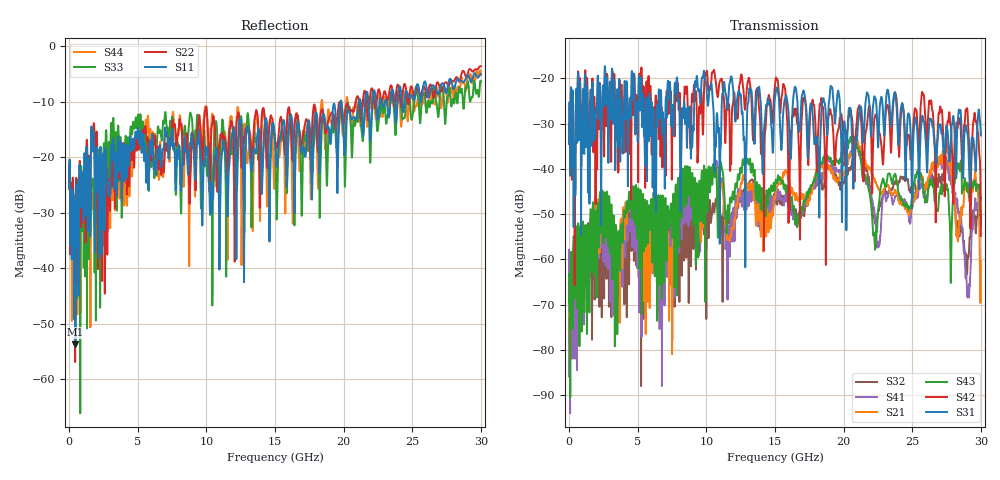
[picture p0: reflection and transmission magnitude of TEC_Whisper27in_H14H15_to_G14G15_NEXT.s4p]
! Tyco Electronics
! H14F15-H14G15_NEXT
!! PART DESCRIPTION: Whisper 27in Megtron 6 VLP-HVLP-VLP Channel Model, bulkhead 2.4mm test pts
!! MODEL DESCRIPTION: System 4-port S-parameter
!! MODEL STATUS: Measured
!! MODEL GEOMETRY: Channel Model
!! MODEL FREQUENCY RANGE: DC to 30.000 GHz in 10.000 MHz frequency steps
!! MODEL EDGE RATE LIMITATION: 12.500 ps (Using conservative 0.5/Fmax rule of thumb)
!! TIME-DOMAIN TRANSFORM CAUTIONS:
!! 1.) Do not simulate transient edge rates faster than the number listed above.  Edge rates faster than this number
!!  contain significant spectral content at frequencies above the model's highest frequency.
!! 2.) Even when simulating edge rates that are slower than the number listed above, be aware that the best time
!!  resolution possible with a direct iFFT is (1 / 2Fmax).  As a result, time resolution is typically not adequate
!!  for most time-domain simulations unless tricks such as windowing are used to minimize leakage and aliasing.
!! 3.) Because the model has a uniform frequency step, a direct iFFT will result in an impulse that that has a time
!!  length given by either (1 / Fstep) or (1 / 2Fstep), depending on the transform being used.  Care has been taken
!!  in selecting the frequency step to ensure a settled impulse response for the model.  Therefore, convolution with
!!  the model's impulse response should present no issues.  However, if directly concatenating s-parameter models
!!  in the frequency domain a user must either interpolate necessary interim frequencies or complete impulse response
!!  zero-padding.  Impulse response zero-padding is more difficult, but more accurate.
!! PORT DEFINITIONS:
!! Port  1  ----->  Side A  H14  G14  Side A  <-----  Port  2
!! Port  3  ----->  Side A  H15  G15  Side A  <-----  Port  4
! Point-to-Point link (differential)  !
! Connectors:  !
!  1: STRADA Whisper  !
! Materials:  !
!  Backplane: Megtron-6 HVLP  !
!  Daughtercard: Megtron-6 VLP  !
! Stack-up:  !
!  Backplane: 20 layers, 200mil thick  !
!  Daughtercard: 14 layers, 110mil thick  !
! Trace Length:  !
!  Backplane: 17in  !
!  Daightercards: 5in  !
! Trace Width:  !
!  Backplane: 8-13-8 mils  !
!  Daughtercards: 6-9-6 mils  !
! Geometry:  !
!  Backplane: Stripline  !
!  Daughtercards: Stripline  !
! Freq. Range: 0 GHz - 30 GHz  !
! Note1: non-mixed-mode s-parameters  !
! Note2: channel includes 2.4mm test points  !
! Touchstone data converted from IdEM dataset
# GHz S MA R 50
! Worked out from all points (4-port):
!   3000 points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, 10 MHz to 30 GHz, reference 50 ohm
!   strongest paths, dB at 10 MHz, 7.51 GHz, 15.01 GHz, 22.51 GHz, 30 GHz:
!     S31: -34.4, -26.1, -24.2, -35.3, -32.6
!     S42: -34.5, -34.3, -21.3, -30.6, -54.8
!     S43: -63.2, -55.2, -44.2, -49.6, -52.4
!     S21: -64.7, -80.9, -46.5, -44.2, -60.4
!     S41: -57.9, -64.9, -45.3, -56.4, -50.4
!     S32: -59.5, -65.0, -47.4, -49.1, -46.5
!   lowest |S11| = -53.7 dB at 470 MHz (marker M1), VSWR 1.00, Z = 50.2 + j0.00336 ohm
!   |S11| at or under -10 dB: start of sweep to 19.78 GHz; 19.83 GHz to 21.11 GHz (1.272 GHz wide, 6.21 % of centre); 21.24 GHz to 21.57 GHz (325.6 MHz wide, 1.52 % of centre)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
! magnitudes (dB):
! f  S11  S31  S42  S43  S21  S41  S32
! 10 MHz  -25.6  -34.4  -34.5  -63.2  -64.7  -57.9  -59.5
! 470 MHz  -53.7  -40.5  -40.2  -53.9  -57.2  -58.6  -57.1
! 20.91 GHz  -13.2  -33.2  -31.2  -33.8  -32.7  -34.4  -33.8
! 22.53 GHz  -12.5  -34.7  -31.0  -48.7  -44.4  -56.2  -49.2
! 27.47 GHz  -8.4  -30.6  -34.0  -43.6  -34.5  -38.2  -37.6
! 29.03 GHz  -5.2  -32.3  -27.3  -44.2  -43.9  -68.4  -60.4
! 30 GHz  -5.0  -32.6  -54.8  -52.4  -60.4  -50.4  -46.5
